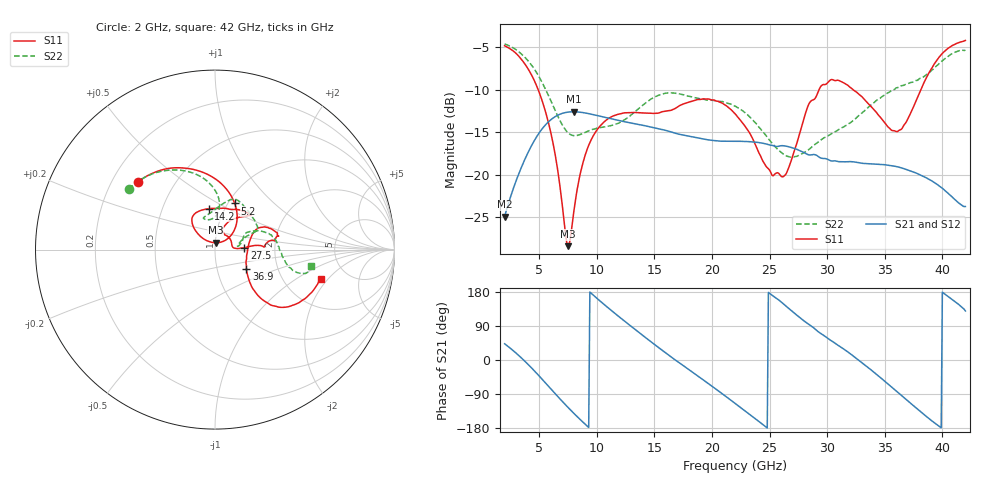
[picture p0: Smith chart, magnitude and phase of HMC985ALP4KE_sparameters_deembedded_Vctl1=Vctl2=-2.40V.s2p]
!s2p File: Measurements: S11, S21, S12, S22
# GHz S dB R 50.0
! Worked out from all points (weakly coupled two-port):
!   401 points, 2 GHz to 42 GHz, reference 50 ohm
!   highest |S21| = -12.59 dB at 8 GHz (marker M1); lowest = -24.9 dB at 2 GHz (marker M2)
!   lowest |S11| = -28.4 dB at 7.5 GHz (marker M3), VSWR 1.08, Z = 50.2 + j3.82 ohm
!   |S11| at or under -10 dB: 4.913 GHz to 29.3 GHz (24.38 GHz wide, 143 % of centre); 32.25 GHz to 38.13 GHz (5.879 GHz wide, 16.7 % of centre)
!   |S22| runs from -17.9 to -4.6 dB; largest |S21 - S12| = 0.00025
!   S11 on the Smith chart (normalised r, x): 2 GHz: 0.31, +0.34; 5.2 GHz: 1.07, +0.60; 14.2 GHz: 0.84, +0.41; 27.5 GHz: 1.39, +0.03; 36.9 GHz: 1.38, -0.31; 42 GHz: 3.22, -1.71
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2  -4.84 138.9  -24.90 42.9  -24.91 42.9  -4.63 145.1
3.6  -6.68 105.2  -18.66 1.4  -18.67 1.4  -5.99 117.9
5.2  -11.07 66.9  -14.70 -48.8  -14.70 -48.8  -9.00 92.7
6.3  -16.96 43.9  -13.24 -85.8  -13.24 -85.8  -12.16 84.1
7.5  -28.37 85.3  -12.63 -125.0  -12.64 -125.0  -15.04 92.1
8  -24.40 129.1  -12.59 -140.4  -12.60 -140.4  -15.39 98.9
8.7  -19.10 137.8  -12.67 -161.1  -12.67 -161.1  -15.19 106.4
10.7  -13.71 128.7  -13.25 144.9  -13.26 144.9  -14.36 107.9
14.2  -12.74 98.8  -14.24 60.0  -14.24 59.9  -11.60 79.3
15.4  -12.73 84.0  -14.61 32.0  -14.61 32.0  -10.63 71.8
19.1  -11.12 45.4  -15.76 -49.4  -15.77 -49.4  -11.13 44.3
22  -12.82 52.3  -16.06 -114.3  -16.07 -114.3  -11.93 24.3
25.3  -20.12 56.6  -16.56 169.1  -16.56 169.1  -16.44 17.8
26.4  -19.95 7.0  -16.62 142.9  -16.62 142.9  -17.73 11.3
27.5  -15.67 3.7  -17.08 115.0  -17.08 115.0  -17.73 8.2
28.7  -11.23 2.9  -17.64 88.1  -17.64 88.1  -16.67 12.4
31.1  -8.98 15.6  -18.46 35.8  -18.46 35.8  -14.61 27.2
33.3  -11.23 26.3  -18.67 -13.7  -18.68 -13.7  -12.42 25.6
35.4  -14.51 6.8  -18.88 -66.3  -18.88 -66.3  -10.29 17.5
36.9  -13.71 -31.9  -19.37 -105.2  -19.38 -105.2  -9.32 8.9
39.7  -6.21 -41.2  -21.27 -174.4  -21.27 -174.6  -6.97 -15.0
42  -4.22 -15.6  -23.72 129.4  -23.73 129.5  -5.35 -9.6
